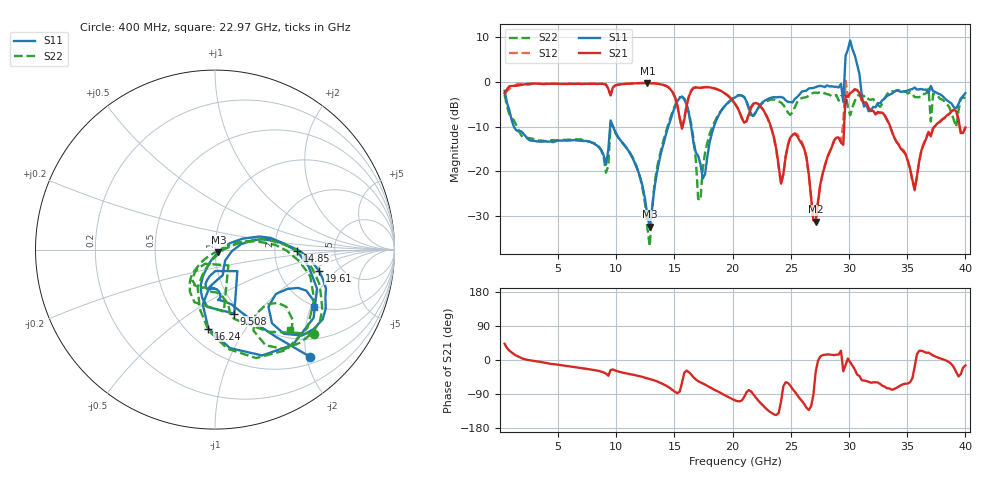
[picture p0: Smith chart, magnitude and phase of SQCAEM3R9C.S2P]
! Network Analyzer HP8722ES.07.66: Jul 25, 2000 Serial No. US39175408
! 26 Oct 2004  14:15:31
! Frequency  S11  S21  S12  S22
# HZ  S  DB R  50
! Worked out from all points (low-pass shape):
!   201 points, 400 MHz to 40 GHz, reference 50 ohm
!   highest |S21| = -0.22 dB at 12.68 GHz (marker M1); lowest = -31.2 dB at 27.13 GHz (marker M2)
!   |S21| within 3 dB of the highest: start of sweep to 15.02 GHz; 16.24 GHz to 19.67 GHz (3.428 GHz wide, 19.1 % of centre)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
!   lowest |S11| = -32.3 dB at 12.87 GHz (marker M3), VSWR 1.05, Z = 51.9 - j1.52 ohm
!   |S11| at or under -10 dB: 1.198 GHz to 9.466 GHz (8.268 GHz wide, 155 % of centre); 9.733 GHz to 14.46 GHz (4.723 GHz wide, 39.1 % of centre); 16.43 GHz to 18.38 GHz (1.95 GHz wide, 11.2 % of centre)
!   |S22| runs from -36.7 to -1.5 dB; largest |S21 - S12| = 0.36
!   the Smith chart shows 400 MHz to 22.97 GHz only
!   S11 on the Smith chart (normalised r, x): 400 MHz: 0.62, -2.07; 9.508 GHz: 0.93, -0.77; 14.85 GHz: 2.68, -0.06; 16.24 GHz: 0.63, -0.69; 19.61 GHz: 3.41, -1.25; 22.97 GHz: 1.95, -2.12
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4e8  -1.94 -48.4  -2.49 43.0  -2.65 47.9  -2.83 -40.5
7.132e9  -13.19 -103.1  -0.41 -21.7  -0.42 -21.9  -13.04 -121.2
9.508e9  -8.59 -73.3  -3.00 -26.6  -2.88 -25.9  -9.14 -81.9
1.2676e10  -30.02 -84.6  -0.22 -48.4  -0.21 -48.3  -32.80 -115.1
1.2874e10  -32.34 -37.3  -0.26 -50.0  -0.22 -50.1  -36.70 -37.8
1.3666e10  -17.90 22.3  -0.44 -58.7  -0.39 -58.7  -17.12 16.8
1.4854e10  -6.80 -1.1  -2.31 -79.8  -2.33 -79.8  -6.46 -7.9
1.624e10  -7.11 -94.8  -3.22 -32.0  -3.10 -31.7  -6.87 -94.4
1.723e10  -18.34 -67.2  -1.31 -59.0  -1.22 -58.7  -26.45 0.1
1.9606e10  -4.55 -11.6  -3.07 -97.5  -3.01 -97.3  -4.69 -14.8
2.02e10  -3.46 -23.6  -4.91 -106.5  -4.85 -106.1  -3.31 -29.0
2.2972e10  -3.89 -30.2  -7.91 -130.8  -7.87 -130.5  -4.24 -47.2
2.6932e10  -1.33 -45.6  -30.90 -93.0  -30.89 -89.8  -2.41 -47.4
2.713e10  -1.14 -45.6  -31.23 -32.3  -31.25 -30.0  -2.35 -49.8
2.9308e10  -0.42 -22.6  -13.56 24.4  -13.37 25.0  -3.14 -40.0
2.9506e10  -4.45 28.7  -14.04 -29.9  -9.26 -15.6  -3.00 67.1
3.01e10  9.30 -66.5  -2.48 -6.1  -2.45 -5.6  -7.45 -62.4
3.0496e10  5.99 -80.7  -1.68 -25.0  -1.57 -23.8  -4.23 -62.4
3.0694e10  3.89 81.5  -1.85 -38.6  -1.77 -37.1  -3.06 118.9
3.1486e10  -5.01 -79.9  -4.57 -55.3  -4.68 -55.6  -3.04 -68.6
3.3466e10  -2.84 -30.9  -9.42 -74.8  -9.54 -74.3  -2.04 -46.7
4e10  -2.49 -60.8  -10.16 -14.1  -10.23 -11.9  -3.63 -34.8
